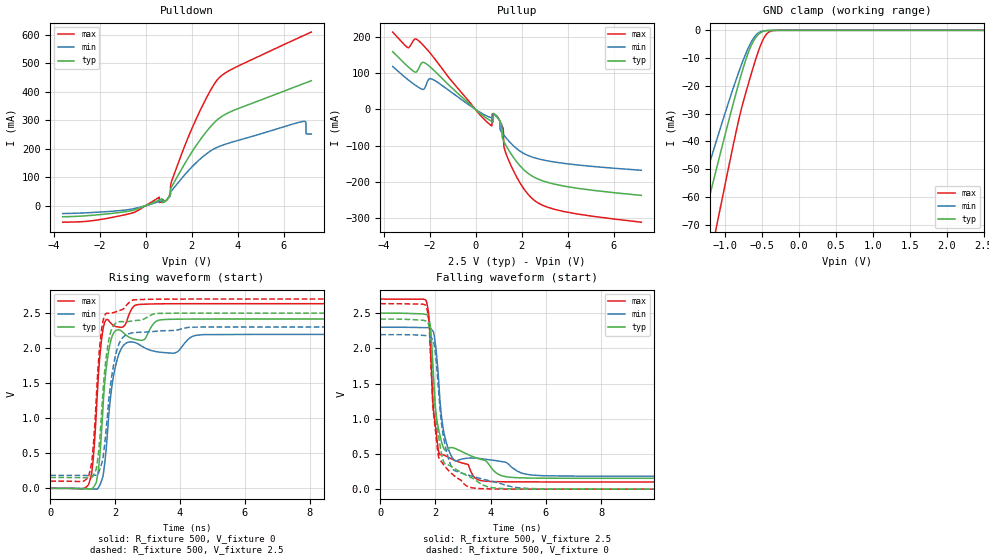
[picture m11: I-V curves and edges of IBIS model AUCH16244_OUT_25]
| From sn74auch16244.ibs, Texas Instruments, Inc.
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[Model]   AUCH16244_OUT_25
Model_type  3-state
Enable   Active-Low
Vref =   0
Rref =   500
Cref =   30p
Vmeas =   1.25
| variable   typ   min   max
C_comp   5.23pF   4.67pF   5.46pF
| C_pullup   7.79pF   4.61pF   11.93pF
| C_pulldown   6.72pF   4.62pF   15.56pF
| C_tri-state   5.23pF   4.67pF   5.46pF
[Temperature Range]   40   100   -40
| Ambient temperature   25   85   -40
[Voltage range]   2.5   2.3   2.7
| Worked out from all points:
|   slope of the pulldown table from 0 to 0.375 V, typ, clamps not added: 30.7 ohm
|   slope of the pullup table from 0 to 0.375 V, typ, clamps not added: 19 ohm
|   GND clamp passes 1 mA (typ) near -0.53 V on its own axis
|   rising waveform, R_fixture 500, V_fixture 0: 20-80 % time 261ps typ, 320ps min, 234ps max; typ from 0 V to 2.42 V
|   falling waveform, R_fixture 500, V_fixture 2.5: 20-80 % time 390ps typ, 388ps min, 280ps max; typ from 2.5 V to 0.154 V
|   rising waveform, R_fixture 500, V_fixture 2.5: 20-80 % time 262ps typ, 329ps min, 231ps max; typ from 0.154 V to 2.5 V
|   falling waveform, R_fixture 500, V_fixture 0: 20-80 % time 359ps typ, 424ps min, 284ps max; typ from 2.42 V to 0 V
[GND Clamp]
| AUCH16244_OUT_25
|   Voltage   I(typ)   I(min)   I(max)
-3.6V     -322.9mA   -271.3mA   -392.8mA
-1.455V   -86.41mA   -69.74mA   -115.3mA
-1.345V   -74.46mA   -59.86mA   -100.9mA
-1.295V   -69.05mA   -55.41mA   -94.31mA
-1.105V   -48.71mA   -38.79mA   -69.37mA
-850mV    -22.51mA   -17.75mA   -36.48mA
-725mV    -11.06mA   -8.768mA   -23.02mA
-625mV    -4.339mA   -3.267mA   -13.84mA
-520mV    -878.8uA   -491uA     -5.429mA
-430mV    -104.5uA   -60.64uA   -1.111mA
-325mV    -4.915uA   -5.536uA   -43.94uA
2.5V      1.045nA    211.8nA    1.502nA
[Pulldown]
| AUCH16244_OUT_25
|   Voltage   I(typ)   I(min)   I(max)
-3.6V     -38.75mA   -27.46mA   -57.79mA
-1.14V    -23.79mA   -17.18mA   -36mA
590mV     19.92mA    14.98mA    30.03mA
600mV     20.28mA    15.25mA    11.17mA
910mV     20.16mA    20.33mA    19.24mA
1.07V     37.88mA    45.66mA    41.07mA
1.915V    176.4mA    127.8mA    252.5mA
3.135V    303.2mA    205.9mA    444mA
6.825V    427.7mA    295.8mA    596.2mA
6.965V    431.9mA    293mA      601.3mA
6.97V     432.1mA    252.7mA    601.5mA
7.2V      439mA      251.9mA    609.9mA
[Pullup]
| AUCH16244_OUT_25
|   Voltage   I(typ)   I(min)   I(max)
-3.6V     160mA      119mA      214.2mA
-2.935V   118.6mA    82.49mA    170.9mA
-2.405V   122.6mA    58.64mA    186.2mA
-1.88V    112.5mA    83.79mA    148.8mA
670mV     -31.69mA   -22.93mA   -44.2mA
720mV     -33.47mA   -24.18mA   -12.23mA
935mV     -20.74mA   -21.43mA   -18.64mA
1.19V     -83.17mA   -67.47mA   -51.41mA
1.235V    -89.46mA   -71.21mA   -103.5mA
1.49V     -117.6mA   -90.51mA   -148.5mA
2.565V    -188.1mA   -133.7mA   -252.1mA
7.2V      -237.7mA   -168.2mA   -311.9mA
[Ramp]
| AUCH16244_OUT_25
| variable   typ   min   max
dV/dt_r   1.46/2.67E-10   1.32/3.25E-10   1.58/2.43E-10
dV/dt_f   1.41/3.99E-10   1.27/3.98E-10   1.56/2.85E-10
R_load = 500
[Rising Waveform]
| AUCH16244_OUT_25
R_fixture =   500
C_fixture =   0
L_fixture =   0
V_fixture =   0
V_fixture_min = 0
V_fixture_max = 0
|   Time   V(typ)   V(min)   V(max)
0s        12.33nV    36.82nV    2.005nV
1.175ns   -8.763mV   -5.395mV   48.9mV
1.325ns   11.49mV    -9.841mV   427.4mV
1.49ns    294.4mV    14.46mV    1.658V
1.66ns    1.403V     288.2mV    2.342V
1.885ns   2.139V     1.405V     2.348V
2.195ns   2.244V     1.998V     2.297V
2.7ns     2.119V     2.062V     2.621V
3.68ns    2.411V     1.93V      2.633V
34.99ns   2.416V     2.195V     2.634V
[Falling Waveform]
| AUCH16244_OUT_25
R_fixture =   500
C_fixture =   0
L_fixture =   0
V_fixture =   2.5
V_fixture_min = 2.3
V_fixture_max = 2.7
|   Time   V(typ)   V(min)   V(max)
0s        2.5V       2.3V       2.7V
1.66ns    2.48V      2.294V     2.681V
1.765ns   2.409V     2.295V     2.452V
1.935ns   1.56V      2.223V     1.105V
2.135ns   813.5mV    1.428V     506.1mV
2.295ns   586.5mV    824.7mV    485.7mV
2.6ns     590.7mV    453.7mV    427mV
3.645ns   423.3mV    433.5mV    122.3mV
5.28ns    158.7mV    212.3mV    103.1mV
34.99ns   154.5mV    184.4mV    102.7mV
[Rising Waveform]
| AUCH16244_OUT_25
R_fixture =   500
C_fixture =   0
L_fixture =   0
V_fixture =   2.5
V_fixture_min = 2.3
V_fixture_max = 2.7
|   Time   V(typ)   V(min)   V(max)
0s        154.5mV    184.4mV    102.6mV
1.175ns   152.8mV    182.5mV    163.2mV
1.31ns    173.7mV    182.8mV    521.6mV
1.46ns    407.4mV    198.8mV    1.633V
1.625ns   1.376V     432.6mV    2.385V
1.725ns   1.873V     853.5mV    2.494V
1.845ns   2.203V     1.432V     2.498V
2.12ns    2.376V     2.063V     2.535V
2.57ns    2.39V      2.22V      2.688V
34.99ns   2.5V       2.3V       2.7V
[Falling Waveform]
| AUCH16244_OUT_25
R_fixture =   500
C_fixture =   0
L_fixture =   0
V_fixture =   0
V_fixture_min = 0
V_fixture_max = 0
|   Time   V(typ)   V(min)   V(max)
0s        2.416V     2.195V     2.634V
1.66ns    2.388V     2.181V     2.606V
1.765ns   2.317V     2.178V     2.37V
1.935ns   1.486V     2.092V     1.057V
2.12ns    735mV      1.373V     449.1mV
2.275ns   412.8mV    776.6mV    357.8mV
2.53ns    331.8mV    364.2mV    242.5mV
3.32ns    159.6mV    184.4mV    19.83mV
5.965ns   567.3uV    3.429mV    109.5uV
34.99ns   29.82uV    1.81uV     13.69uV
